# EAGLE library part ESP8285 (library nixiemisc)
The ESP8285
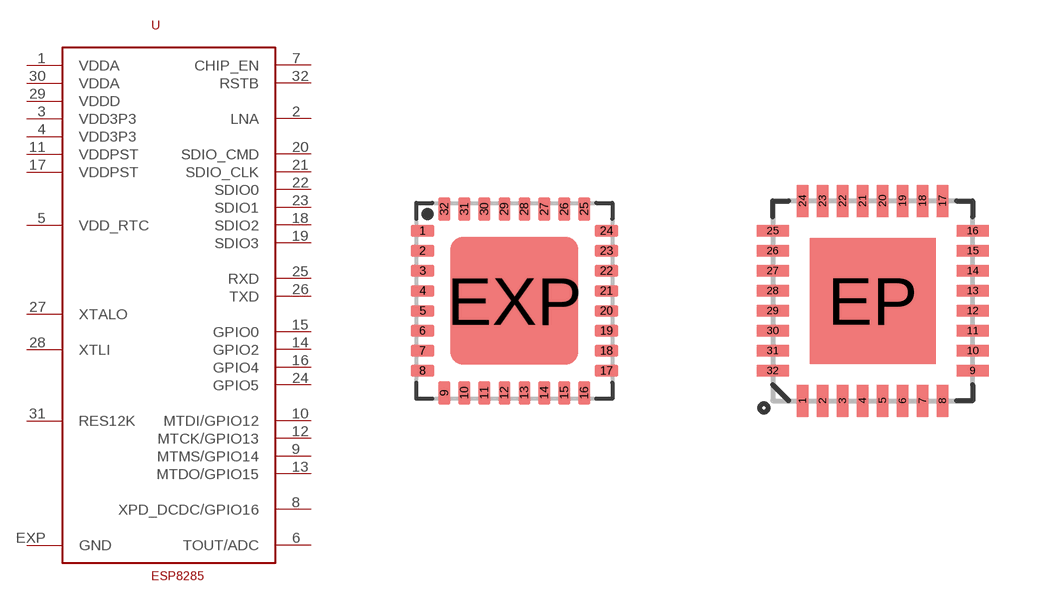
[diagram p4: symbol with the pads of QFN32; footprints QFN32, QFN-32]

Designator prefix U

## ESP8285QFN32  [QFN32]
1  VDDA  pwr
2  LNA
3  VDD3P3  pwr
4  VDD3P3  pwr
5  VDD_RTC  nc
6  TOUT/ADC  in
7  CHIP_EN  in
8  XPD_DCDC/GPIO16
9  MTMS/GPIO14
10  MTDI/GPIO12
11  VDDPST  pwr
12  MTCK/GPIO13
13  MTDO/GPIO15
14  GPIO2
15  GPIO0
16  GPIO4
17  VDDPST  pwr
18  SDIO2
19  SDIO3
20  SDIO_CMD
21  SDIO_CLK
22  SDIO0
23  SDIO1
24  GPIO5
25  RXD
26  TXD
27  XTALO
28  XTLI
29  VDDD  pwr
30  VDDA  pwr
31  RES12K  in
32  RSTB  in
EXP  GND  pwr

## ESP8285PHYSICALSYMBOL  [QFN32]
Pads as for QFN32

## ESP8285QFN-32  [QFN-32]
1  VDDA  pwr
2  LNA
3  VDD3P3  pwr
4  VDD3P3  pwr
5  VDD_RTC  nc
6  TOUT/ADC  in
7  CHIP_EN  in
8  XPD_DCDC/GPIO16
9  MTMS/GPIO14
10  MTDI/GPIO12
11  VDDPST  pwr
12  MTCK/GPIO13
13  MTDO/GPIO15
14  GPIO2
15  GPIO0
16  GPIO4
17  VDDPST  pwr
18  SDIO2
19  SDIO3
20  SDIO_CMD
21  SDIO_CLK
22  SDIO0
23  SDIO1
24  GPIO5
25  RXD
26  TXD
27  XTALO
28  XTLI
29  VDDD  pwr
30  VDDA  pwr
31  RES12K  in
32  RSTB  in
EP  GND  pwr

## Footprint QFN32 (pad centres in mm)
QFN 32 Source: http://www.ftdichip.com/Documents/DataSheets/DS_FT232R_v104.pdf
smd 0.6 x 0.3: 1 -2.3,1.75; 2 -2.3,1.25; 3 -2.3,0.75; 4 -2.3,0.25; 5 -2.3,-0.25; 6 -2.3,-0.75; 7 -2.3,-1.25; 8 -2.3,-1.75; 17 2.3,-1.75; 18 2.3,-1.25; 19 2.3,-0.75; 20 2.3,-0.25; 21 2.3,0.25; 22 2.3,0.75; 23 2.3,1.25; 24 2.3,1.75
smd 0.3 x 0.6: 9 -1.75,-2.3; 10 -1.25,-2.3; 11 -0.75,-2.3; 12 -0.25,-2.3; 13 0.25,-2.3; 14 0.75,-2.3; 15 1.25,-2.3; 16 1.75,-2.3; 25 1.75,2.3; 26 1.25,2.3; 27 0.75,2.3; 28 0.25,2.3; 29 -0.25,2.3; 30 -0.75,2.3; 31 -1.25,2.3; 32 -1.75,2.3
smd 3.2 x 3.2: EXP 0,0

## Footprint QFN-32 (pad centres in mm)
QFN 32-Pin package w/ Thermal Pad ***Unproven*** Applicable Parts: TLC5940
smd 0.285 x 0.8: 1 -1.75,-2.5; 2 -1.25,-2.5; 3 -0.75,-2.5; 4 -0.25,-2.5; 5 0.25,-2.5; 6 0.75,-2.5; 7 1.25,-2.5; 8 1.75,-2.5; 17 1.75,2.5; 18 1.25,2.5; 19 0.75,2.5; 20 0.25,2.5; 21 -0.25,2.5; 22 -0.75,2.5; 23 -1.25,2.5; 24 -1.75,2.5
smd 0.8 x 0.285: 9 2.5,-1.75; 10 2.5,-1.25; 11 2.5,-0.75; 12 2.5,-0.25; 13 2.5,0.25; 14 2.5,0.75; 15 2.5,1.25; 16 2.5,1.75; 25 -2.5,1.75; 26 -2.5,1.25; 27 -2.5,0.75; 28 -2.5,0.25; 29 -2.5,-0.25; 30 -2.5,-0.75; 31 -2.5,-1.25; 32 -2.5,-1.75
smd 3.15 x 3.15: EP 0,0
